ORGANIZATION_BLOCK "MAIN"
TITLE =MAIN BLOCK
AUTHOR : Esposito
FAMILY : EGAL_srl
NAME : MAIN
VERSION : 0.1


VAR_TEMP
  OB1_EV_CLASS : BYTE ;	//Bits 0-3 = 1 (Coming event), Bits 4-7 = 1 (Event class 1)
  OB1_SCAN_1 : BYTE ;	//1 (Cold restart scan 1 of OB 1), 3 (Scan 2-n of OB 1)
  OB1_PRIORITY : BYTE ;	//1 (Priority of 1 is lowest)
  OB1_OB_NUMBR : BYTE ;	//1 (Organization block 1, OB1)
  OB1_RESERVED_1 : BYTE ;	//Reserved for system
  OB1_RESERVED_2 : BYTE ;	//Reserved for system
  OB1_PREV_CYCLE : INT ;	//Cycle time of previous OB1 scan (milliseconds)
  OB1_MIN_CYCLE : INT ;	//Minimum cycle time of OB1 (milliseconds)
  OB1_MAX_CYCLE : INT ;	//Maximum cycle time of OB1 (milliseconds)
  OB1_DATE_TIME : DATE_AND_TIME ;	//Date and time OB1 started
END_VAR
BEGIN
NETWORK
TITLE =BIT ALWAYS OFF
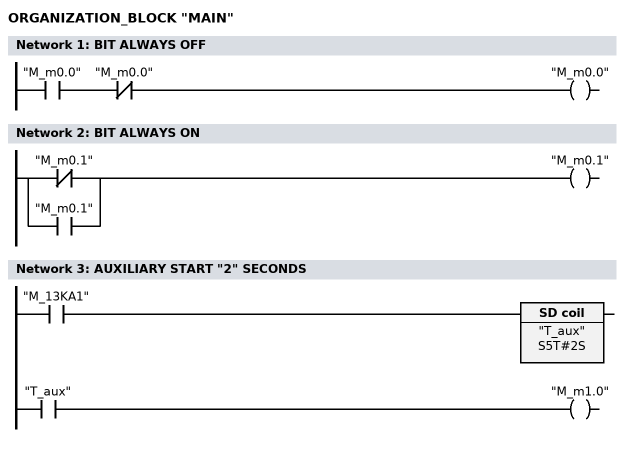
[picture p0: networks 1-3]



      U     "M_m0.0";
      UN    "M_m0.0";
      =     "M_m0.0";
NETWORK
TITLE =BIT ALWAYS ON

      ON    "M_m0.1";
      O     "M_m0.1";
      =     "M_m0.1";
NETWORK
TITLE =AUXILIARY START "2" SECONDS

      U     "M_13KA1";
      L     S5T#2S;
      SE    "T_aux";
      NOP   0;
      NOP   0;
      NOP   0;
      U     "T_aux";
      =     "M_m1.0";
NETWORK
TITLE =AUXILIARY START "5" SECONDS

      U     "M_13KA1";
      =     L     20.0;
      U     L     20.0;
      L     S5T#5S;
      SE    "T_aux_five";
      NOP   0;
      NOP   0;
      NOP   0;
      U     "T_aux_five";
      =     "M_m0.4";
      U     L     20.0;
      U     "M_m0.4";
      FP    "M_m21.7";
      S     "M_m27.0";
NETWORK
TITLE =ORDER LOADED DATA FOR MODULE CAMS
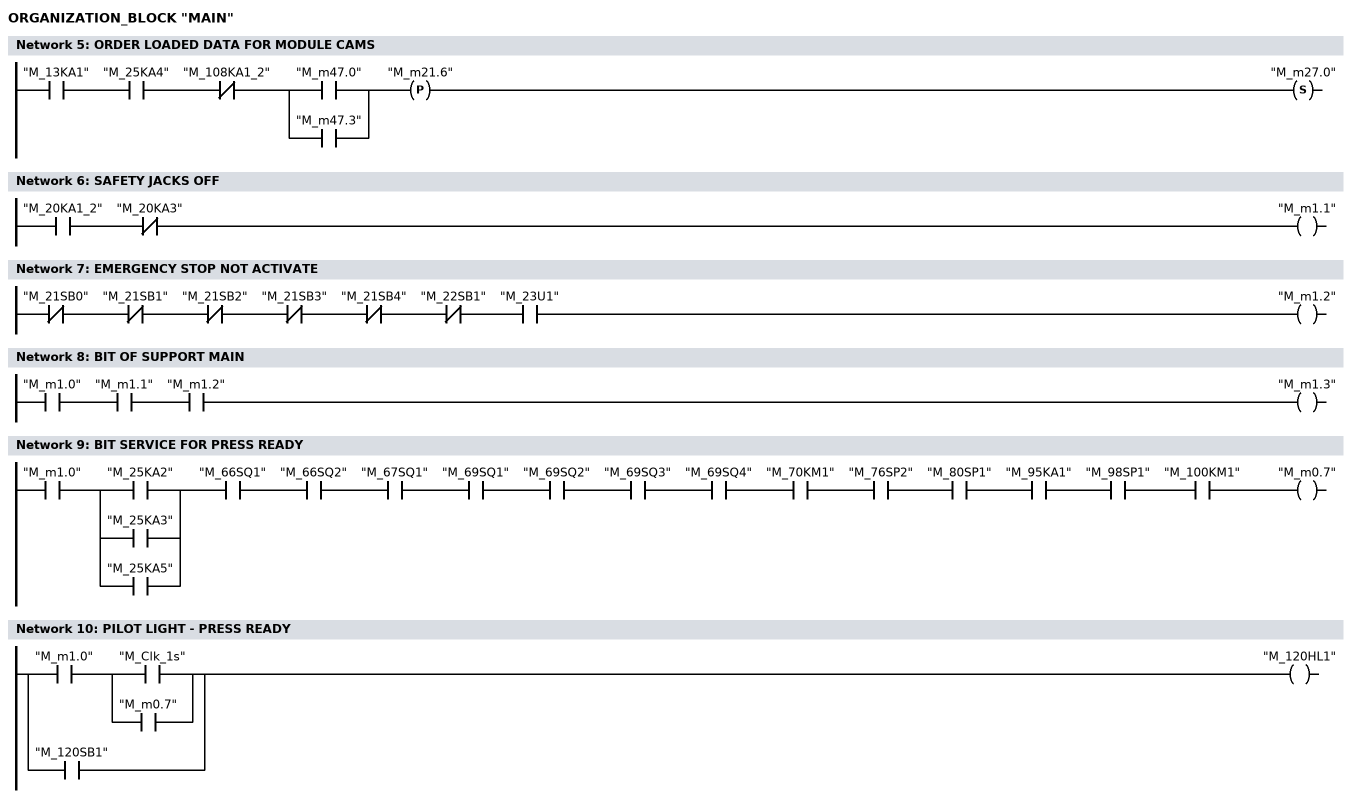
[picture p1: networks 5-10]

      U     "M_13KA1";
      U     "M_25KA4";
      UN    "M_108KA1_2";
      U(    ;
      O     "M_m47.0";
      O     "M_m47.3";
      )     ;
      FP    "M_m21.6";
      S     "M_m27.0";
NETWORK
TITLE =SAFETY JACKS OFF



      U     "M_20KA1_2";
      UN    "M_20KA3";
      =     "M_m1.1";
NETWORK
TITLE =EMERGENCY STOP NOT ACTIVATE



      UN    "M_21SB0";
      UN    "M_21SB1";
      UN    "M_21SB2";
      UN    "M_21SB3";
      UN    "M_21SB4";
      UN    "M_22SB1";
      U     "M_23U1";
      =     "M_m1.2";
NETWORK
TITLE =BIT OF SUPPORT MAIN

      U     "M_m1.0";
      U     "M_m1.1";
      U     "M_m1.2";
      =     "M_m1.3";
NETWORK
TITLE =BIT SERVICE FOR PRESS READY

      U     "M_m1.0";
      U(    ;
      O     "M_25KA2";
      O     "M_25KA3";
      O     "M_25KA5";
      )     ;
      U     "M_66SQ1";
      U     "M_66SQ2";
      U     "M_67SQ1";
      U     "M_69SQ1";
      U     "M_69SQ2";
      U     "M_69SQ3";
      U     "M_69SQ4";
      U     "M_70KM1";
      U     "M_76SP2";
      U     "M_80SP1";
      U     "M_95KA1";
      U     "M_98SP1";
      U     "M_100KM1";
      =     "M_m0.7";
NETWORK
TITLE =PILOT LIGHT - PRESS READY

      U     "M_m1.0";
      U(    ;
      O     "M_Clk_1s";
      O     "M_m0.7";
      )     ;
      O     "M_120SB1";
      =     "M_120HL1";
NETWORK
TITLE =CALL BLOCK FC 20

      UC    FC    20;

NETWORK
TITLE =CALL BLOCK FC 15

      UC    "HANDLING_PROGRAM";

NETWORK
TITLE =CALL BLOCK FC 16

      U     "M_m1.0";
      CC    "WG_SOFT";
NETWORK
TITLE =CALL BLOCK FC 21

      U     "M_m1.0";
      UN    "M_m20.4";
      CC    "ANGLE";
NETWORK
TITLE =CALL FC 24

      UC    "ROBOT_INRFACE";

NETWORK
TITLE =CALL FC 25

      UC    "ROBOT_INRFACE1";

NETWORK
TITLE =CALL BLOCK FC 26

      UC    "PERIPHERAL";

NETWORK
TITLE =CALL BLOCK FC 28

      UC    "TD_17PRESS";

NETWORK
TITLE =CALL BLOCK FC 30



      UC    "ALARM";
NETWORK
TITLE =Call Block 36 Contapezzi

      UC    "TOT_PEZZI";

NETWORK
TITLE =CALL BLOCK FC 37

      UC    "CAMS_PRESS";

NETWORK
TITLE =CALL BLOCK FC 38

      U     "M_m1.0";
      U     "M_m27.0";
      CC    "CAMS_ELECTR";
NETWORK
TITLE =CALL BLOCK FC 65

      UC    "MOV_BOL";

NETWORK
TITLE =CALL BLOCK FC 69

      UC    "CLAMPS";

NETWORK
TITLE =CALL BLOCK FC 70

      UC    "LUBR";

NETWORK
TITLE =CALL FC 75

      UC    "OVERLOAD";

NETWORK
TITLE =CALL FC 76

      UC    "OVERLOAD_M";

NETWORK
TITLE =CALL BLOCK FC 80

      UC    "BALAN";

NETWORK
TITLE =CALL BLOCK FC 85

      UC    "SLIDE";

NETWORK
TITLE =CALL BLOCK FC 95

      UC    "MAIN_MOT";

NETWORK
TITLE =CALL BLOCK FC 96

      UC    FC    96;

NETWORK
TITLE =CALL BLOCK FC 100

      UC    "TORC_PAC";

NETWORK
TITLE =CALL BLOCK FC 109

      UC    "CLUTCH";

NETWORK
TITLE =CALL BLOCK FC 114

      UC    "CONVEYOR";

NETWORK
TITLE =CALL BLOCK FC 115

      UC    "DIE_ALARM";

NETWORK
TITLE =CALL BLOCK FC 116

      UC    "SCRAPES_CUTES";

NETWORK
TITLE =CALL BLOCK FC 117

      UC    "INLETS";

NETWORK
TITLE =CALL BLOCK FC 118

      UC    "CO_DB_DB";

NETWORK
TITLE =CALL BLOCK FC 119

      UC    "STATUS_OP_DB";

END_ORGANIZATION_BLOCK

